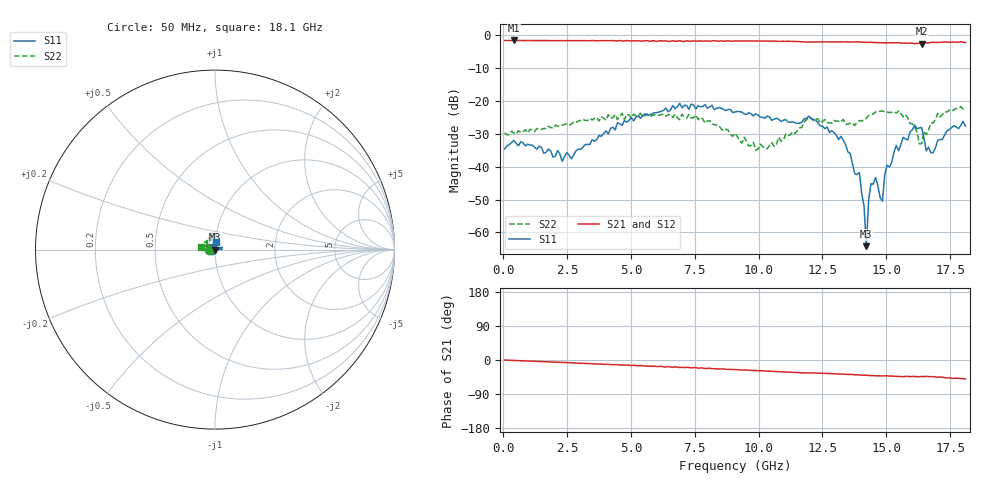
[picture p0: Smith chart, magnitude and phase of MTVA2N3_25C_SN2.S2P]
! Network Analyzer HP8720D.06.14 Serial No. US36140669
! 11 May 2005  12:36:15
! Frequency  S11  S21  S12  S22
# HZ  S  DB R 50
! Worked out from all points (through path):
!   201 points, 50 MHz to 18.1 GHz, reference 50 ohm
!   highest |S21| = -1.66 dB at 411 MHz (marker M1); lowest = -2.6 dB at 16.39 GHz (marker M2)
!   group delay of S21, straight-line fit = 7.6 ps
!   lowest |S11| = -64.2 dB at 14.22 GHz (marker M3), VSWR 1.00, Z = 50 + j0.0448 ohm
!   |S11| at or under -10 dB: start of sweep to end of sweep
!   |S22| runs from -35.0 to -21.8 dB; largest |S21 - S12| = 0.026
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5e7  -34.63 -173.4  -1.68 -0.2  -1.70 -0.7  -29.68 -175.6
4.11e8  -32.06 -175.0  -1.66 -1.3  -1.66 -1.6  -29.84 179.6
2.30625e9  -38.41 154.1  -1.72 -6.6  -1.71 -6.9  -27.40 157.7
3.1185e9  -34.07 107.8  -1.72 -8.8  -1.72 -9.4  -25.64 153.2
6.09675e9  -23.38 91.5  -1.78 -17.1  -1.72 -17.3  -24.39 112.9
9.075e9  -23.42 116.7  -1.82 -25.4  -1.80 -25.8  -29.90 109.5
1.03385e10  -24.64 130.1  -1.84 -29.3  -1.84 -29.9  -34.53 148.4
1.21435e10  -25.67 133.5  -2.14 -33.8  -2.11 -34.4  -26.03 140.3
1.32265e10  -30.80 126.2  -2.12 -37.1  -2.12 -37.6  -26.38 135.6
1.39485e10  -41.76 138.5  -2.16 -39.5  -2.12 -40.1  -26.00 154.2
1.4129e10  -51.87 138.7  -2.17 -40.1  -2.15 -40.7  -25.71 154.3
1.421925e10  -64.17 46.4  -2.25 -40.3  -2.23 -40.9  -25.33 159.5
1.43095e10  -50.30 -103.4  -2.23 -40.8  -2.18 -41.5  -24.48 155.3
1.439975e10  -45.21 -95.8  -2.21 -41.0  -2.20 -41.3  -24.30 153.3
1.458025e10  -43.31 -97.8  -2.31 -41.7  -2.21 -42.2  -23.39 152.0
1.4851e10  -50.51 76.2  -2.39 -42.1  -2.32 -42.4  -23.09 143.2
1.494125e10  -42.41 26.2  -2.37 -41.8  -2.41 -41.9  -23.35 143.0
1.512175e10  -40.13 11.3  -2.38 -42.3  -2.30 -42.4  -23.56 137.2
1.57535e10  -31.60 22.8  -2.46 -43.4  -2.56 -44.7  -24.21 119.9
1.638525e10  -28.12 -1.7  -2.63 -43.5  -2.49 -43.9  -33.06 148.5
1.674625e10  -35.77 45.5  -2.30 -44.2  -2.34 -44.7  -26.70 179.0
1.81e10  -27.68 83.7  -2.32 -49.9  -2.26 -51.5  -22.24 168.9
